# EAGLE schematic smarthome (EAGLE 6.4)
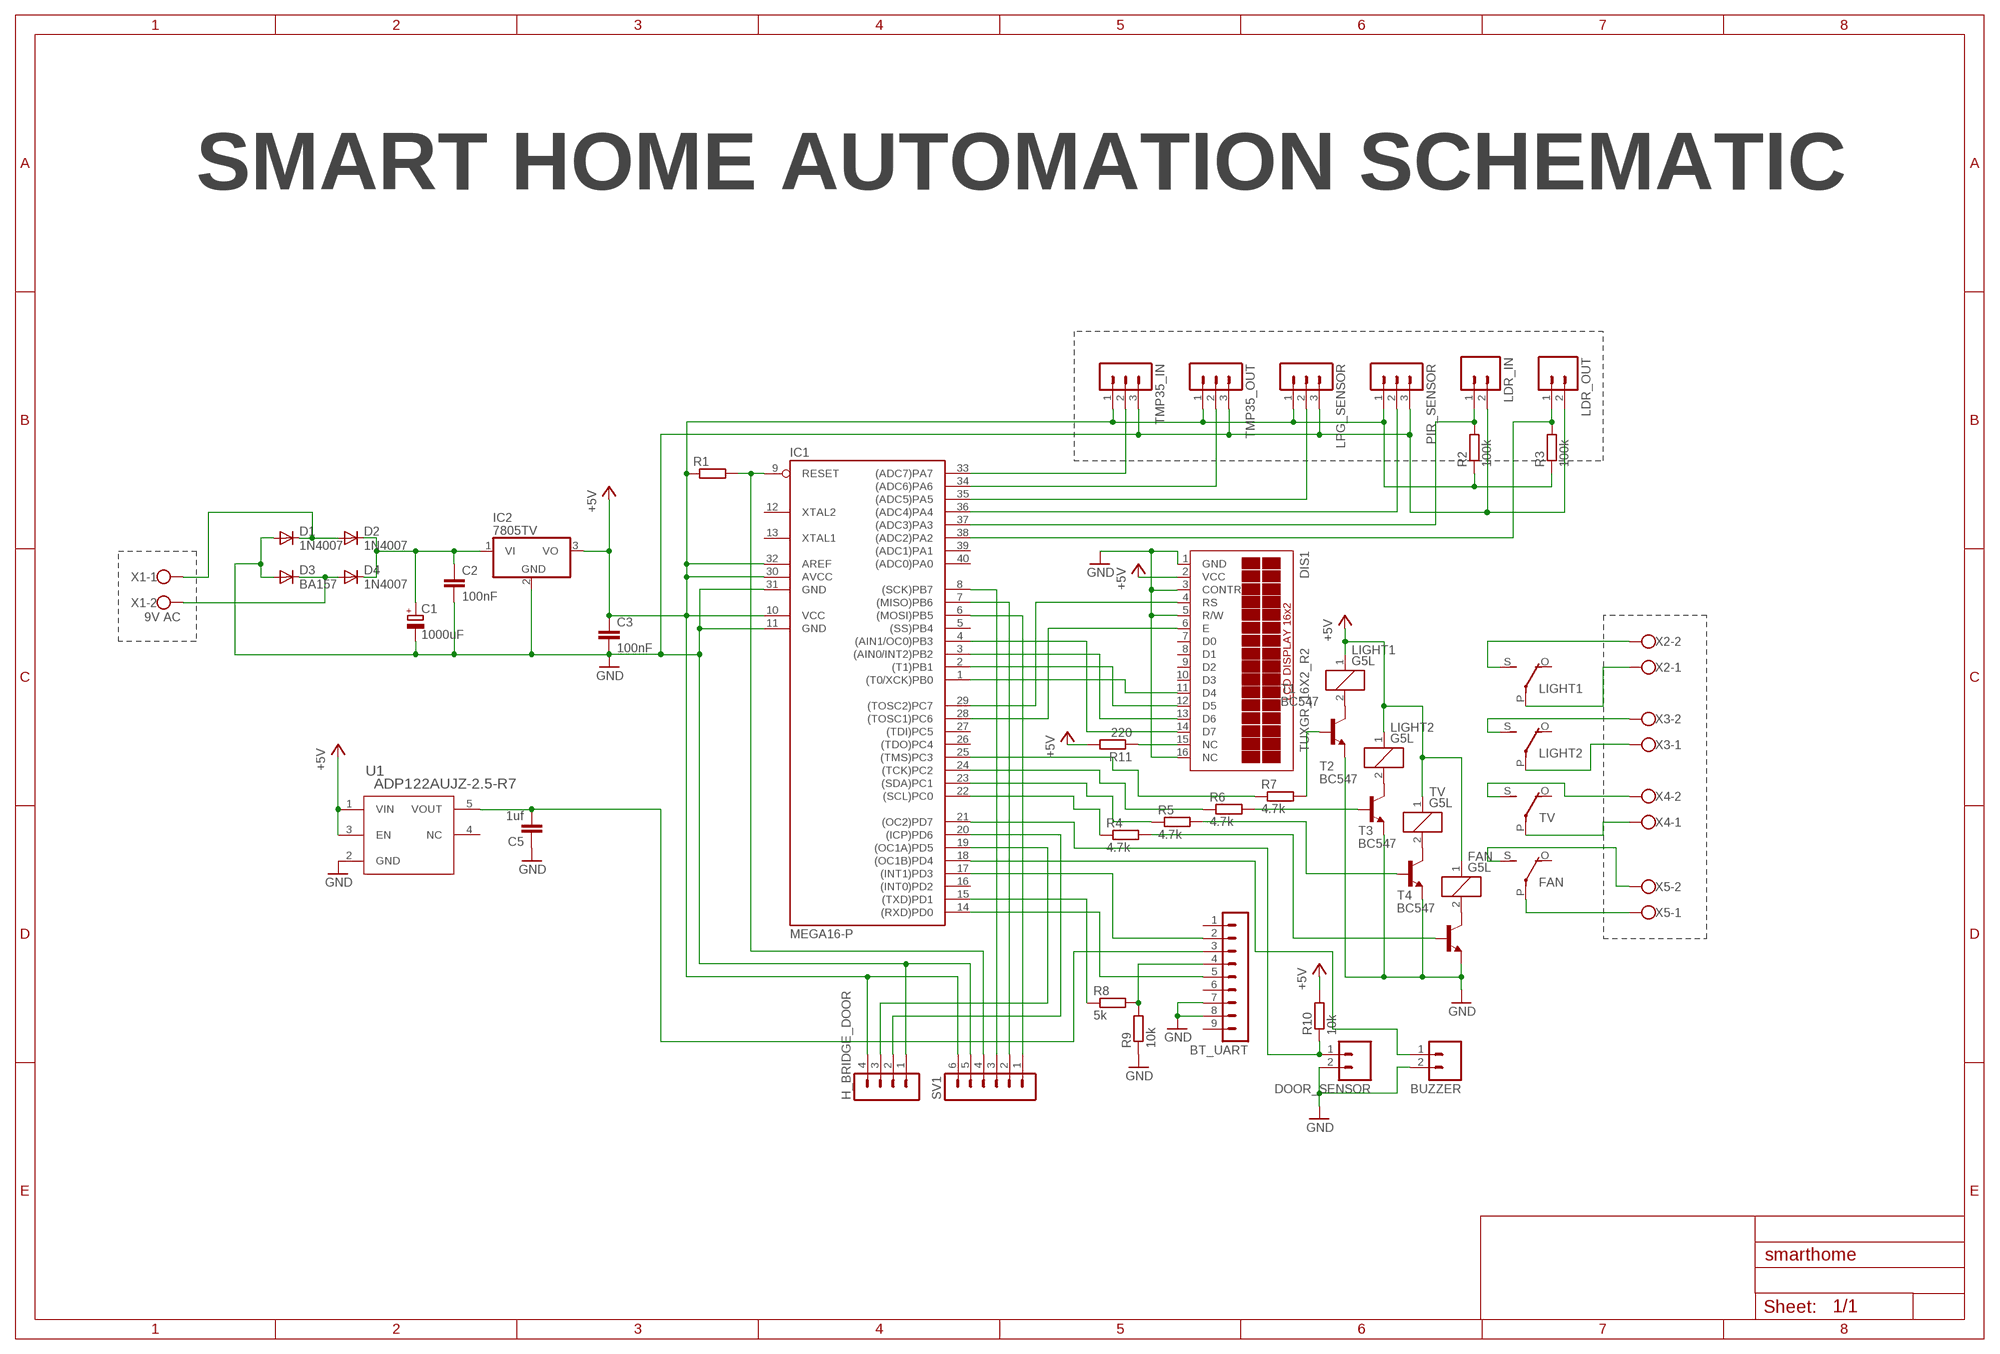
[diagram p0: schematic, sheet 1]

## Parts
BT_UART  MA09-1  [MA09-1]
BUZZER  M02  [02P]
C1  1000uF  CPOL-EUE3.5-8  [E3,5-8]
C2  100nF  C-EU050-055X075  [C050-055X075]
C3  100nF  C-EU050-055X075  [C050-055X075]
C5  1uf  C-EU050-035X075  [C050-035X075]
D1  1N4007  BA157  [P1-10]
D2  1N4007  BA157  [P1-10]
D3  BA157  [P1-10]
D4  1N4007  BA157  [P1-10]
DIS1  TUXGR_16X2_R2  [TUXGR_16X2_R2]
DOOR_SENSOR  M02  [02P]
FAN  G5L  [G5LE]
H_BRIDGE_DOOR  MA04-1  [MA04-1]
IC1  MEGA16-P  [DIL40]
IC2  7805TV  [TO220V]
LDR_IN  M02  [02P]
LDR_OUT  M02  [02P]
LIGHT1  G5L  [G5LE]
LIGHT2  G5L  [G5LE]
LPG_SENSOR  MA03-1  [MA03-1]
PIR_SENSOR  MA03-1  [MA03-1]
R1  R-EU_0309/10  [0309/10]
R2  100k  R-EU_0309/10  [0309/10]
R3  100k  R-EU_0309/10  [0309/10]
R4  4.7k  R-EU_0309/10  [0309/10]
R5  4.7k  R-EU_0309/10  [0309/10]
R6  4.7k  R-EU_0309/10  [0309/10]
R7  4.7k  R-EU_0309/10  [0309/10]
R8  5k  R-EU_0309/10  [0309/10]
R9  10k  R-EU_0309/10  [0309/10]
R10  10k  R-EU_0309/10  [0309/10]
R11  220  R-EU_0309/10  [0309/10]
SV1  MA06-1  [MA06-1]
T1  BC547  [TO92]
T2  BC547  [TO92]
T3  BC547  [TO92]
T4  BC547  [TO92]
TMP35_IN  MA03-1  [MA03-1]
TMP35_OUT  MA03-1  [MA03-1]
TV  G5L  [G5LE]
U1  ADP122AUJZ-2.5-R7  [UJ_5]
X1  9V AC  W237-102  [W237-102]
X2  W237-102  [W237-102]
X3  W237-102  [W237-102]
X4  W237-102  [W237-102]
X5  W237-102  [W237-102]

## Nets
+5V: C3.1 DIS1.2(VCC) FAN.1 H_BRIDGE_DOOR.4 IC1.10(VCC) IC1.30(AVCC) IC1.32(AREF) IC2.3(VO) LIGHT1.1 LIGHT2.1 LPG_SENSOR.1 PIR_SENSOR.1 R1.1 R2.1 R3.1 R10.2 R11.2 SV1.6 TMP35_IN.1 TMP35_OUT.1 TV.1 U1.1(VIN) U1.3(EN)
GND: BT_UART.7 BT_UART.8 BUZZER.2 C1.- C2.2 C3.2 C5.1 D1.A D3.A DIS1.1(GND) DIS1.5(R/W) DIS1.16(NC) DOOR_SENSOR.2 H_BRIDGE_DOOR.1 IC1.11(GND) IC1.31(GND) IC2.2(GND) LDR_IN.2 LDR_OUT.2 LPG_SENSOR.3 PIR_SENSOR.3 R9.1 SV1.5 T1.1(E) T2.1(E) T3.1(E) T4.1(E) TMP35_IN.3 TMP35_OUT.3 U1.2(GND)
N$1: D1.C D2.A X1.1
N$2: D3.C D4.A X1.2
N$3: BT_UART.5 IC1.14((RXD)PD0)
N$4: C1.+ C2.1 D2.C D4.C IC2.1(VI)
N$5: BT_UART.4 R8.2 R9.2
N$6: IC1.9(RESET) R1.2 SV1.4
N$7: IC1.37((ADC3)PA3) LDR_IN.1 R2.2
N$8: IC1.38((ADC2)PA2) LDR_OUT.1 R3.2
N$9: IC1.33((ADC7)PA7) TMP35_IN.2
N$10: IC1.34((ADC6)PA6) TMP35_OUT.2
N$11: IC1.35((ADC5)PA5) LPG_SENSOR.2
N$12: IC1.36((ADC4)PA4) PIR_SENSOR.2
N$13: IC1.22((SCL)PC0) R4.1
N$14: IC1.23((SDA)PC1) R5.1
N$15: IC1.24((TCK)PC2) R6.1
N$16: IC1.25((TMS)PC3) R7.1
N$17: R7.2 T1.2(B)
N$18: R6.2 T2.2(B)
N$19: R5.2 T3.2(B)
N$20: R4.2 T4.2(B)
N$21: LIGHT1.2 T1.3(C)
N$22: LIGHT2.2 T2.3(C)
N$23: T3.3(C) TV.2
N$24: FAN.2 T4.3(C)
N$25: IC1.15((TXD)PD1) R8.1
N$26: BT_UART.2 IC1.17((INT1)PD3)
N$27: DOOR_SENSOR.1 IC1.21((OC2)PD7) R10.1
N$28: DIS1.6(E) IC1.28((TOSC1)PC6)
N$29: DIS1.4(RS) IC1.29((TOSC2)PC7)
N$30: DIS1.14(D7) IC1.4((AIN1/OC0)PB3)
N$31: DIS1.13(D6) IC1.3((AIN0/INT2)PB2)
N$32: DIS1.12(D5) IC1.2((T1)PB1)
N$33: DIS1.11(D4) IC1.1((T0/XCK)PB0)
N$34: IC1.6((MOSI)PB5) SV1.1
N$35: BUZZER.1 IC1.18((OC1B)PD4)
N$36: IC1.7((MISO)PB6) SV1.2
N$37: IC1.8((SCK)PB7) SV1.3
N$38: H_BRIDGE_DOOR.2 IC1.20((ICP)PD6)
N$39: H_BRIDGE_DOOR.3 IC1.19((OC1A)PD5)
N$40: LIGHT1.P(2:P) X2.1
N$41: LIGHT1.S(2:S) X2.2
N$42: LIGHT2.P(2:P) X3.1
N$43: LIGHT2.S(2:S) X3.2
N$44: TV.S(2:S) X4.2
N$45: TV.P(2:P) X4.1
N$46: FAN.S(2:S) X5.2
N$47: FAN.P(2:P) X5.1
N$48: DIS1.15(NC) R11.1
N$49: BT_UART.3 C5.2 U1.5(VOUT)
Unconnected: BT_UART.1 BT_UART.6 BT_UART.9 DIS1.3(CONTR) DIS1.7(D0) DIS1.8(D1) DIS1.9(D2) DIS1.10(D3) FAN.O(2:O) IC1.5((SS)PB4) IC1.12(XTAL2) IC1.13(XTAL1) IC1.16((INT0)PD2) IC1.26((TDO)PC4) IC1.27((TDI)PC5) IC1.39((ADC1)PA1) IC1.40((ADC0)PA0) LIGHT1.O(2:O) LIGHT2.O(2:O) TV.O(2:O) U1.4(NC)

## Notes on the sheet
- SMART HOME AUTOMATION SCHEMATIC

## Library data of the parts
BT_UART = con-lstb:MA09-1: PIN HEADER; OC_FARNELL: unknown; OC_NEWARK: unknown
BUZZER DOOR_SENSOR LDR_IN LDR_OUT = con-amp-quick:M02: AMP QUICK CONNECTOR; OC_FARNELL: unknown; OC_NEWARK: unknown
C1 = resistor:CPOL-EU: POLARIZED CAPACITOR, European symbol
C2 C3 C5 = resistor:C-EU: CAPACITOR, European symbol
D1-D4 = diode:BA157: DIODE
DIS1 = display-lcd:TUXGR_16X2_R2: Tuxgraphics LCD display 16x2 characters reflective, without background light Source: tuxgr_12x2_r2.pdf; OC_FARNELL: unknown; OC_NEWARK: unknown
FAN LIGHT1 LIGHT2 TV = relay:G5L: RELAY 1 x switch, 10 A/120 V AC, 8 A/30 V ADC, Omron; OC_FARNELL: unknown; OC_NEWARK: unknown
H_BRIDGE_DOOR = con-lstb:MA04-1: PIN HEADER; OC_FARNELL: unknown; OC_NEWARK: unknown
IC1 = atmel:MEGA16-P: MICROCONTROLLER 16 Kbytes FLASH 1 kbytes SRAM 512 bytes EEPROM USART 8-channel 10 bit ADC Source: avr.lbr; MPN: ATMEGA16-16PU; OC_FARNELL: 9171142; OC_NEWARK: 01M6885
IC2 = linear:78*: Positive VOLTAGE REGULATOR Source: http://cache.national.com/ds/LM/LM78L05.pdf http://www.fairchildsemi.com/ds/LM/LM7805.pdf
LPG_SENSOR PIR_SENSOR TMP35_IN TMP35_OUT = con-lstb:MA03-1: PIN HEADER; OC_FARNELL: unknown; OC_NEWARK: unknown
R1-R11 = resistor:R-EU_: RESISTOR, European symbol
SV1 = con-lstb:MA06-1: PIN HEADER; OC_FARNELL: unknown; OC_NEWARK: unknown
T1-T4 = transistor:BC547: NPN TRANSISTOR
U1 = ADP122:ADP122AUJZ-2.5-R7
X1-X5 = con-wago-500:W237-102: WAGO SCREW CLAMP; MPN: 237-102; OC_FARNELL: unknown; OC_NEWARK: 70K9898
